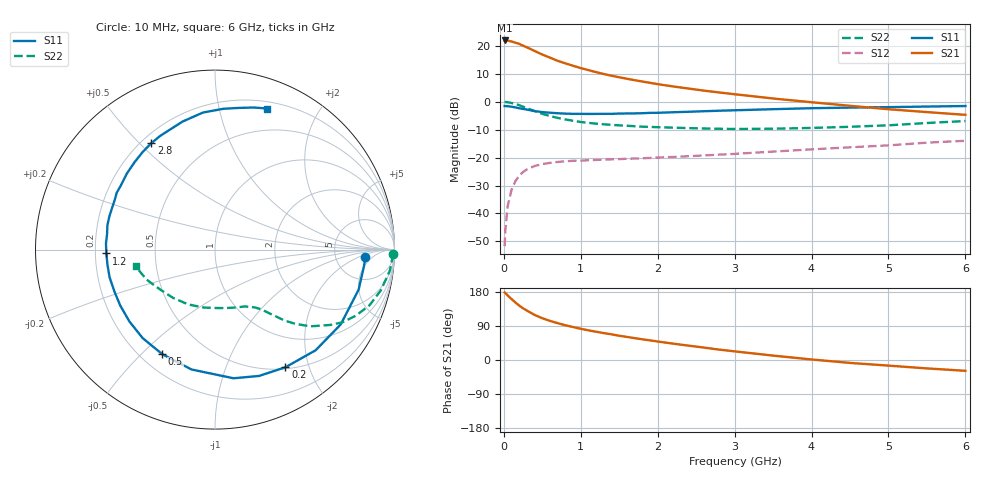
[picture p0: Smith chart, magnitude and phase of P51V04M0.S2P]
! SIEMENS Small Signal Semiconductors
! BFP183
! Si NPN RF Bipolar Junction Transistor in SOT143
! VCE = 1 V  IC = 4 mA
! Common Emitter S-Parameters:  March  1996
# GHz  S  MA  R  50
!  f  S11  S21  S12  S22
! GHz  MAG  ANG  MAG  ANG  MAG  ANG  MAG  ANG
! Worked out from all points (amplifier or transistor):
!   36 points, 10 MHz to 6 GHz, reference 50 ohm
!   highest |S21| = 21.9 dB at 10 MHz (marker M1)
!   |S21| within 3 dB of that: start of sweep to 341 MHz
!   unconditionally stable (mu >= 1): 1.615 GHz to end of sweep
!   at 250 MHz: K = 0.19, MSG = 22.6 dB, |S12| = -25.2 dB
!   at 1.4 GHz: K = 0.91, MSG = 15.0 dB, |S12| = -20.6 dB
!   at 6 GHz: K = 1.02, MAG = 3.7 dB, |S12| = -14.0 dB
!   S11 on the Smith chart (normalised r, x): 10 MHz: 10, -3; 200 MHz: 0.52, -1.64; 500 MHz: 0.29, -0.58; 1.2 GHz: 0.25, -0.02; 2.8 GHz: 0.24, +0.54; 6 GHz: 0.27, +1.41
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0.01  0.8388 -3.0  12.51 178.3  0.0026 88.9  0.9939 -1.4
0.02  0.8353 -6.3  12.41 176.6  0.0051 86.2  0.9891 -2.9
0.05  0.8307 -15.6  12.43 170.3  0.0136 83.6  0.981 -6.9
0.1  0.8151 -30.8  11.98 160.8  0.0265 73.0  0.9515 -13.8
0.15  0.7931 -45.0  11.41 151.9  0.0378 66.6  0.9152 -19.8
0.2  0.764 -59.1  10.87 143.6  0.0478 60.4  0.8673 -25.1
0.25  0.7455 -70.8  10.08 136.4  0.0551 54.5  0.8165 -29.8
0.3  0.7243 -81.8  9.406 130.4  0.0616 49.7  0.7669 -33.2
0.4  0.6806 -101.1  8.119 118.9  0.0707 42.3  0.6808 -38.9
0.5  0.6526 -116.8  6.993 110.2  0.0766 36.5  0.6083 -42.8
0.6  0.6368 -129.3  6.158 103.2  0.0806 32.8  0.5545 -45.5
0.7  0.6227 -140.0  5.406 97.2  0.0837 30.0  0.5138 -47.2
0.8  0.613 -149.5  4.87 91.6  0.0859 27.6  0.4824 -48.7
1.1  0.605 -172.0  3.683 78.2  0.0899 24.1  0.418 -52.5
1.2  0.6058 -178.0  3.386 74.6  0.0909 23.1  0.4058 -53.8
1.6  0.6169 162.5  2.58 60.9  0.0954 22.2  0.3722 -58.9
2.2  0.6486 139.2  1.879 43.2  0.1028 22.9  0.3439 -69.5
2.8  0.6911 120.9  1.467 27.4  0.1131 23.9  0.3284 -82.9
3.5  0.736 104.2  1.144 11.6  0.1281 23.7  0.3291 -101.1
4.5  0.7859 86.6  0.846 -7.7  0.153 20.9  0.3563 -131.0
5.5  0.8207 74.7  0.653 -22.2  0.1853 16.9  0.4165 -156.4
6  0.8384 69.6  0.583 -28.5  0.2003 13.0  0.4518 -168.0
